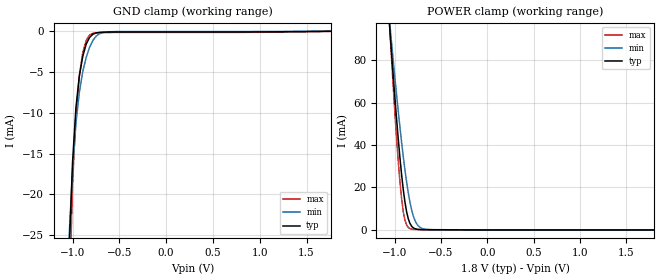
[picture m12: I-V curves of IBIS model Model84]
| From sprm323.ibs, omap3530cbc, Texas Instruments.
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| Model based on original model for IQ0120CS_7LM
|   Sub model IQ0120CS_7LM_PU_ON_1P8
[model]   Model84
|[Input Load]   PU
|[Output Drive]
|Voltage   1.8V
|Mode   INPUT
Model_type   Input
Polarity   Non-Inverting
Vinl =  0.63
Vinh =  1.17
C_comp   0.4946683p   0.3869884p   0.6246171p
[Model Spec]
Vinl   0.63   0.567   0.6615
Vinh   1.17   1.053   1.2285
[Temperature Range]   25   125   -40
[Voltage Range]   1.8   1.62   1.89
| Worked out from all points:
|   GND clamp passes 1 mA (typ) near -0.83 V on its own axis
|   POWER clamp passes 1 mA (typ) near -0.80 V on its own axis
[POWER_clamp]
-1.8V     607.9mA    493.5mA    734.7mA
-1.055V   94.78mA    97.3mA     95.12mA
-1.036V   83.8mA     88.72mA    81.51mA
-981.8mV  52.72mA    63.99mA    43.75mA
-945.5mV  34.39mA    48.68mA    23.04mA
-927.3mV  26.31mA    41.49mA    14.92mA
-890.9mV  13.23mA    28.37mA    4.694mA
-836.4mV  3.085mA    13.09mA    637.8uA
-800mV    993.9uA    6.568mA    271.9uA
-763.6mV  371.7uA    2.94mA     199.6uA
-654.5mV  121.2uA    238.2uA    157.2uA
1.8V      4.664nA    2.125nA    7.754nA
[GND_clamp]
-1.8V     -542.2mA   -381.9mA   -758.2mA
-1.036V   -27.01mA   -25.18mA   -34.07mA
-1V       -16.07mA   -17.03mA   -18.75mA
-963.6mV  -9.368mA   -11.28mA   -10.23mA
-927.3mV  -5.476mA   -7.472mA   -5.465mA
-890.9mV  -3.09mA    -4.96mA    -2.629mA
-854.5mV  -1.598mA   -3.225mA   -1.129mA
-818.2mV  -762.5uA   -1.975mA   -471.3uA
-781.8mV  -370.4uA   -1.111mA   -253.8uA
-745.5mV  -205.8uA   -579.8uA   -197.4uA
-600mV    -107.3uA   -67.88uA   -157.9uA
1.764V    -5.54uA    14.03uA    -26.2uA
